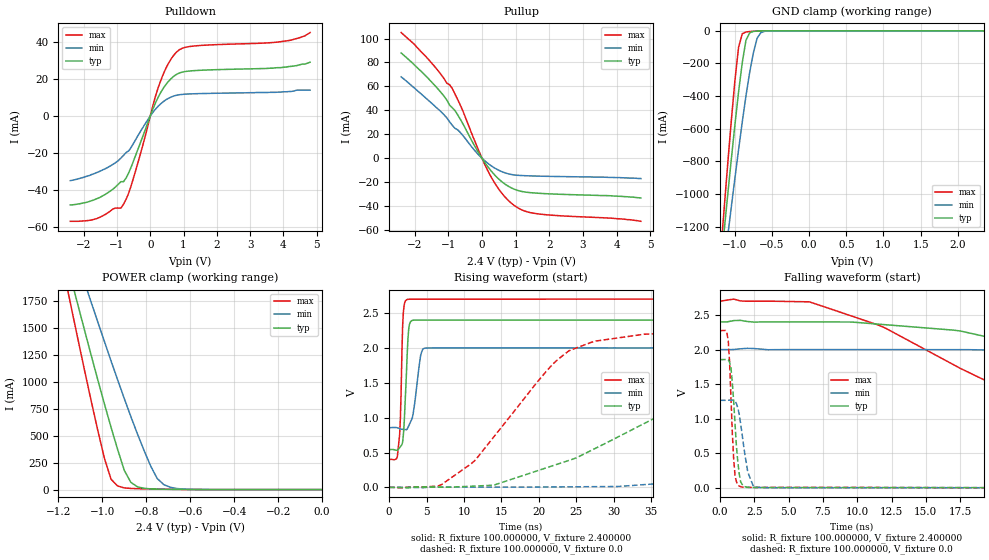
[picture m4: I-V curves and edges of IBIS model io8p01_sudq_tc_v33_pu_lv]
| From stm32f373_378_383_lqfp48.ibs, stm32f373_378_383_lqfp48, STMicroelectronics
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|   Model io8p01_sudq_tc_v33_pu_lv
[Model]  io8p01_sudq_tc_v33_pu_lv
Model_type I/O
Polarity   Non-Inverting
Enable   Active-Low
Vinl =   0.720000V
Vinh =   1.680000V
Vmeas =  1.200000V
Cref =   50.000000pF
Rref =   100.000000M
Vref =   0.0V
C_comp   1.373400pF   1.288200pF   1.481900pF
[Temperature Range]   25.000000   0.125000k   -40.000000
[Pullup Reference]   2.400000V   2.000000V   2.700000V
[Pulldown Reference]   0.0V   0.0V   0.0V
[POWER Clamp Reference]   2.400000V   2.000000V   2.700000V
[GND Clamp Reference]   0.0V   0.0V   0.0V
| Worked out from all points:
|   slope of the pulldown table from 0 to 0.36 V, typ, clamps not added: 25.7 ohm
|   slope of the pullup table from 0 to 0.36 V, typ, clamps not added: 26.8 ohm
|   GND clamp passes 1 mA (typ) near -0.67 V on its own axis
|   POWER clamp passes 1 mA (typ) near -0.60 V on its own axis
|   rising waveform, R_fixture 100.000000, V_fixture 2.400000: 20-80 % time 460ps typ, 800ps min, 337ps max; typ from 0.543 V to 2.4 V
|   rising waveform, R_fixture 100.000000, V_fixture 0.0: 20-80 % time 22.3ns typ, 64.5ns min, 10.4ns max; typ from 0.001 V to 1.86 V
|   falling waveform, R_fixture 100.000000, V_fixture 2.400000: 20-80 % time 28.8ns typ, 66ns min, 14.6ns max; typ from 2.4 V to 0.543 V
|   falling waveform, R_fixture 100.000000, V_fixture 0.0: 20-80 % time 390ps typ, 567ps min, 290ps max; typ from 1.86 V to 0.001 V
[Pulldown]
|Voltage   I(typ)   I(min)   I(max)
-2.4V     -47.9mA    -34.8mA    -56.7mA
-1.6V     -44.5mA    -30.4mA    -55.2mA
-880mV    -35.33mA   -22.63mA   -49.55mA
-800mV    -35.33mA   -21.13mA   -47.42mA
-640mV    -30.33mA   -18.65mA   -41.16mA
-480mV    -23.12mA   -14mA      -31.94mA
240mV     10.22mA    5.339mA    15.38mA
480mV     17.22mA    8.864mA    26.1mA
800mV     22.59mA    11.27mA    34.68mA
1.28V     24.44mA    12mA       37.7mA
4.16V     26.7mA     13.2mA     40.7mA
4.8V      29mA       14mA       45mA
[Pullup]
|Voltage   I(typ)   I(min)   I(max)
-2.4V     88mA       68mA       105mA
-2V       77.8mA     58.5mA     95mA
-1.36V    59.6mA     42.5mA     75.1mA
-880mV    42.12mA    27.44mA    58.22mA
-560mV    28.45mA    18.75mA    39mA
-160mV    7.44mA     4.66mA     10.64mA
160mV     -6.607mA   -3.947mA   -9.704mA
480mV     -16.91mA   -9.806mA   -25.1mA
880mV     -24.89mA   -13.63mA   -37.75mA
1.2V      -27.87mA   -14.5mA    -43.37mA
1.6V      -29.13mA   -14.89mA   -46.24mA
4.72V     -33.2mA    -17mA      -52.7mA
[GND_clamp]
|Voltage   I(typ)   I(min)   I(max)
-2.4V     -7.358A    -6.372A    -8.78A
-1.2V     -1.489A    -1.65A     -1.416A
-1.15V    -1.254A    -1.461A    -1.124A
-1.1V     -1.024A    -1.273A    -838.2mA
-1.05V    -797.6mA   -1.088A    -563.1mA
-950mV    -374.6mA   -728.7mA   -100.8mA
-900mV    -194.3mA   -557.9mA   -18.01mA
-850mV    -56.94mA   -397.4mA   -7.08mA
-750mV    -3.582mA   -133.8mA   -2.771mA
-700mV    -1.516mA   -44.7mA    -1.516mA
-600mV    -235.4uA   -2.939mA   -209.5uA
2.35V     0A         0A         0A
[POWER_clamp]
|Voltage   I(typ)   I(min)   I(max)
-2.4V     9.979A     9.967A     9.901A
-1.17V    2.182A     2.481A     1.978A
-1.14V    1.945A     2.294A     1.683A
-1.11V    1.71A      2.108A     1.391A
-1.08V    1.476A     1.923A     1.102A
-1.05V    1.245A     1.739A     819.9mA
-960mV    578.3mA    1.196A     96.08mA
-900mV    179.5mA    846.7mA    16.05mA
-870mV    67.19mA    678.8mA    10.83mA
-780mV    6.763mA    219.9mA    5.868mA
-720mV    3.368mA    46.35mA    3.823mA
0V        0A         0A         0A
[Ramp]
| variable   typ   min   max
dV/dt_r  1.11291/22.26359n   0.75672/64.50243n   1.36532/10.38649n
dV/dt_f  1.11417/28.71603n   0.68433/66.27145n   1.37899/14.59538n
R_load = 100.000000
[Rising Waveform]
R_fixture= 100.000000
V_fixture= 2.400000
V_fixture_min= 2.000000
V_fixture_max= 2.700000
|time   V(typ)   V(min)   V(max)
0s        543.1mV    857mV      401.7mV
1.101ns   530.8mV    855mV      448.7mV
1.502ns   584.3mV    840.1mV    998.7mV
1.802ns   651.1mV    832.8mV    2.324V
1.902ns   757.9mV    831.8mV    2.514V
2.402ns   1.893V     834.6mV    2.694V
2.803ns   2.366V     927.3mV    2.699V
4.204ns   2.4V       1.893V     2.699V
4.705ns   2.4V       1.995V     2.699V
49.85ns   2.4V       2V         2.7V
[Rising Waveform]
R_fixture= 100.000000
V_fixture= 0.0
V_fixture_min= 0.0
V_fixture_max= 0.0
|time   V(typ)   V(min)   V(max)
0s        956.5uV    1.197mV    860.5uV
7.007ns   5.369mV    4.197mV    41.39mV
11.51ns   19.97mV    4.204mV    392.1mV
21.02ns   282mV      6.543mV    1.668V
24.02ns   388.1mV    8.718mV    1.96V
34.03ns   914.8mV    40.08mV    2.196V
47.55ns   1.542V     143.3mV    2.258V
64.56ns   1.771V     324.4mV    2.271V
139.1ns   1.856V     1.13V      2.276V
249.2ns   1.856V     1.267V     2.276V
[Falling Waveform]
R_fixture= 100.000000
V_fixture= 2.400000
V_fixture_min= 2.000000
V_fixture_max= 2.700000
|time   V(typ)   V(min)   V(max)
0s        2.4V       2V         2.7V
6.507ns   2.4V       2V         2.691V
17.52ns   2.269V     2V         1.729V
27.03ns   1.852V     1.972V     882.8mV
36.04ns   1.476V     1.914V     536.1mV
54.05ns   856.4mV    1.689V     438.5mV
71.57ns   641.8mV    1.466V     410.8mV
105.1ns   567.6mV    1.136V     401.1mV
152.2ns   545.8mV    929.7mV    401.7mV
249.2ns   543.1mV    857mV      401.7mV
[Falling Waveform]
R_fixture= 100.000000
V_fixture= 0.0
V_fixture_min= 0.0
V_fixture_max= 0.0
|time   V(typ)   V(min)   V(max)
0s        1.856V     1.267V     2.276V
600.6ps   1.852V     1.268V     2.134V
800.8ps   1.733V     1.271V     1.294V
1.001ns   1.237V     1.266V     404.7mV
1.101ns   911.4mV    1.252V     168.6mV
1.301ns   372.2mV    1.155V     45.26mV
1.602ns   54.48mV    790.5mV    12.74mV
2.102ns   8.689mV    187.4mV    7.675mV
2.803ns   5.667mV    8.277mV    7.617mV
49.85ns   956.5uV    1.197mV    860.5uV
